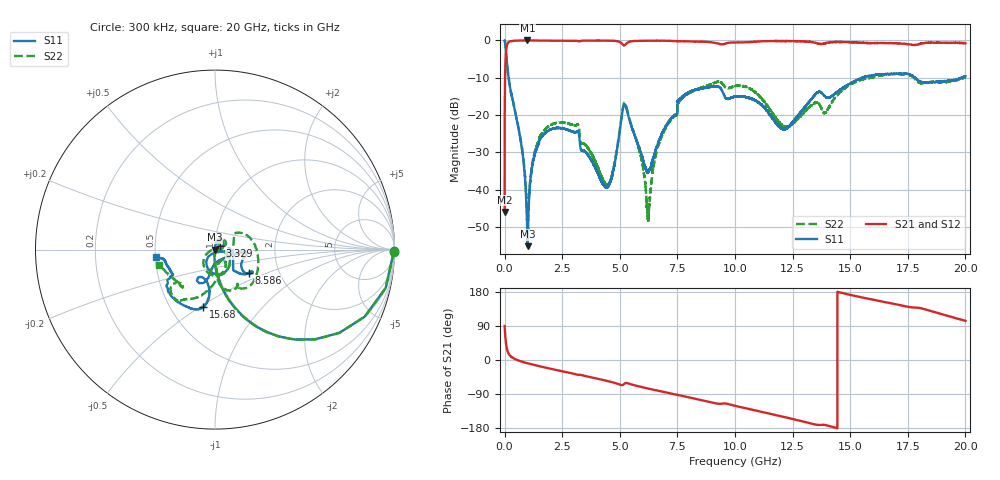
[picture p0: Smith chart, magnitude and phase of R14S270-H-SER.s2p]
!{R14S270}
!Johanson Technology Inc.
!www.johansontechnology.com
!Test Board Conditions:
!Substrate Type  RO4350B
!Substrate Thickness  20 mil
!Substrate Dk  3.66
!TL Type: GCPW
!TL Trace Width  36 mil
!TL Gap  12 mil
!Electrode orientation  Horizontal
!DUT TOPOLOGY	SERIES
!Mounting Pad LxW  26x36 mil
! Created Wed Nov 25 17:33:21 2020
! 2 Port Network Data from SP1.SP block
! freq  magS11  angS11  magS21  angS21  magS12  angS12  magS22  angS22
# khz S ma R 50
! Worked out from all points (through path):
!   20001 points, 300 kHz to 20 GHz, reference 50 ohm
!   highest |S21| = 0.00 dB at 993.3 MHz (marker M1); lowest = -46.0 dB at 300 kHz (marker M2)
!   group delay of S21, straight-line fit = 35.7 ps
!   lowest |S11| = -55.2 dB at 995.3 MHz (marker M3), VSWR 1.00, Z = 49.8 + j0.00131 ohm
!   |S11| at or under -10 dB: 173.2 MHz to 15.51 GHz (15.34 GHz wide, 196 % of centre); 17.82426 GHz to 17.82585 GHz (1.587 MHz wide, 0.00891 % of centre); 17.83 GHz to 19.83 GHz (2.007 GHz wide, 10.7 % of centre)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
!   |S22| runs from -49.6 to 0.0 dB; largest |S21 - S12| = 0.021
!   S11 on the Smith chart (normalised r, x): 300 kHz: open; 3.329 GHz: 1.05, +0.04; 8.586 GHz: 1.40, -0.38; 15.68 GHz: 0.72, -0.52; 20 GHz: 0.50, -0.05
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300  0.9967 -0.5  0.004999 89.9  0.005065 89.9  0.9962 -0.7
137300  0.3908 -68.0  0.9179 21.8  0.9187 21.7  0.3927 -68.0
738300  0.03774 -95.3  0.9984 -4.2  0.9982 -4.2  0.03909 -91.5
993300  0.00207 -173.3  0.9996 -8.7  0.9986 -8.7  0.0035 -24.9
995300  0.001739 179.6  0.9991 -8.8  0.9984 -8.7  0.003357 -20.1
1257300  0.02538 84.4  0.9981 -12.9  0.9984 -12.9  0.0272 65.4
1662300  0.05335 73.5  0.9955 -18.6  0.9952 -18.6  0.05915 67.6
3329300  0.03362 38.6  0.9883 -39.6  0.9881 -39.6  0.04153 36.5
3334300  0.03348 39.1  0.9885 -39.7  0.9892 -39.7  0.04157 37.4
4497300  0.01121 10.3  0.9939 -56.0  0.9932 -55.9  0.01134 16.6
5237300  0.1359 -88.5  0.8752 -61.0  0.8758 -61.0  0.1423 -96.2
5906300  0.03139 -126.5  0.9898 -70.7  0.9895 -70.8  0.02816 -163.5
6234300  0.01739 -73.6  0.9925 -75.4  0.992 -75.4  0.003909 113.4
6667300  0.04258 -15.6  0.9915 -81.2  0.9913 -81.3  0.03811 17.0
7600300  0.1644 -47.5  0.9762 -93.3  0.9759 -93.2  0.1543 37.2
8586300  0.2279 -34.7  0.9607 -106.5  0.9592 -106.5  0.2338 -2.3
1.00003e7  0.1753 -9.8  0.9398 -120.8  0.9388 -120.9  0.2439 -60.8
1.21523e7  0.06411 -66.7  0.9804 -150.8  0.9824 -150.6  0.06969 -63.7
1.33343e7  0.1655 -104.1  0.9498 -168.2  0.9522 -168.2  0.1359 -73.0
1.56773e7  0.3284 -101.8  0.9259 163.2  0.9284 163.1  0.3072 -116.7
1.66673e7  0.3525 -114.1  0.9237 150.9  0.9144 150.7  0.3543 -125.7
2e7  0.3318 -172.5  0.9188 103.3  0.9173 103.7  0.3218 -164.5
